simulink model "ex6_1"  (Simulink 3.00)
settings: Solver=FixedStepDiscrete  SolverMode=SingleTasking  StartTime=0.0  StopTime=100.0  RelTol=1e-3  AbsTol=1e-6

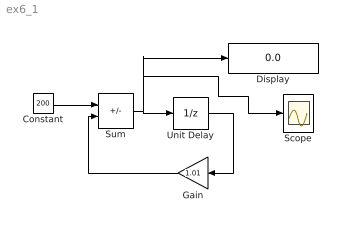
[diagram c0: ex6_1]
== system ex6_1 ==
  Constant : Constant  Value=200
  Display : Display
  Gain : Gain  Orientation=left  Gain=1.01  SaturateOnIntegerOverflow=on
  Scope : Scope
  Sum : Sum  Inputs=-+  SaturateOnIntegerOverflow=on
  Unit Delay : UnitDelay  X0=15000  SampleTime=1
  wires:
  Constant/1 -> Sum/1
  Gain/1 -> Sum/2
  Sum/1 -> Unit Delay/1, Display/1, Scope/1
  Unit Delay/1 -> Gain/1
